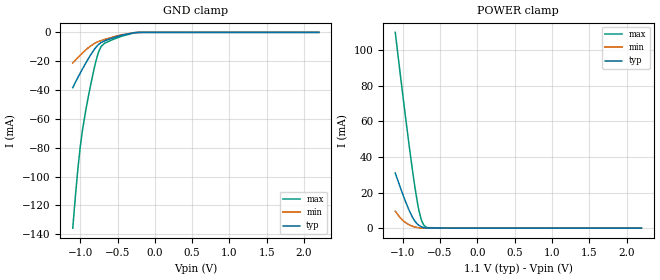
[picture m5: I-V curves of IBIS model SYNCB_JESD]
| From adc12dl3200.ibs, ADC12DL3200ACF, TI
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|   Model SYNCB_JESD
[Model]   SYNCB_JESD
Model_type   Input
Vinl = .57
Vinh = 1.33
|   (nom PVT)   (fast PVT)   (slow PVT)
|   typ   min   max
C_comp   0.804p   0.760p   0.851p
[Voltage Range]   1.1   1.05   1.15
[Temperature Range]   27   125   -40
[Power Clamp Reference]   1.1   1.05   1.15
[GND Clamp Reference]   0   0   0
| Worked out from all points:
|   GND clamp passes 1 mA (typ) near -0.35 V on its own axis
|   POWER clamp passes 1 mA (typ) near -0.76 V on its own axis
[GND Clamp]
|   Voltage   I(typ)   I(min)   I(max)
-1.1V     -38.35mA   -21.26mA   -135.8mA
-1.031V   -31.21mA   -17.49mA   -94.47mA
-1.001V   -28.34mA   -15.93mA   -80.05mA
-968mV    -25.21mA   -14.25mA   -67.2mA
-928.4mV  -21.56mA   -12.32mA   -54.89mA
-862.4mV  -15.8mA    -9.467mA   -37.05mA
-786.5mV  -10.18mA   -7.057mA   -19.36mA
-720.5mV  -7.098mA   -5.706mA   -9.867mA
-674.3mV  -5.925mA   -4.944mA   -7.56mA
-436.7mV  -1.925mA   -1.597mA   -2.529mA
-222.2mV  -53.71uA   -55.81uA   -83.38uA
2.2V      0A         0A         0A
[POWER Clamp]
|   Voltage   I(typ)   I(min)   I(max)
-1.1V     30.96mA    9.496mA    110mA
-1.037V   23.42mA    6.048mA    88.02mA
-964.7mV  15.2mA     3.207mA    63.2mA
-911.9mV  9.817mA    1.854mA    45.83mA
-872.3mV  6.379mA    1.116mA    33.45mA
-836mV    3.901mA    624.7uA    22.9mA
-789.8mV  1.806mA    247.6uA    11.45mA
-753.5mV  844.2uA    105.5uA    5.111mA
-720.5mV  359.1uA    46.09uA    1.923mA
-684.2mV  119.2uA    18.69uA    528.2uA
-275mV    1.918uA    1.014uA    5.44uA
2.2V      0A         0A         0A
